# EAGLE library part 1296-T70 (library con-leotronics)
1.27mm SINGLE ROW FEMALE SOCKET Source: http://www.leotronics.co.uk/Conexcon/Data%20Sheets/sec.%20A/1296ing.pdf
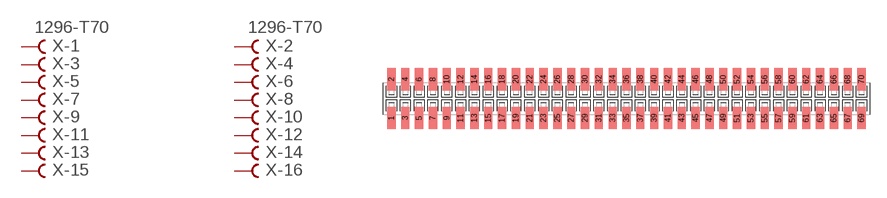
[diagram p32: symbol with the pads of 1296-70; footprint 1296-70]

Designator prefix X; gates -1=FVAL -2=FVAL -3=F -4=F -5=F -6=F -7=F -8=F -9=F -10=F -11=F -12=F -13=F -14=F -15=F -16=F -17=F -18=F -19=F -20=F -21=F -22=F -23=F -24=F -25=F -26=F -27=F -28=F -29=F -30=F -31=F -32=F -33=F -34=F -35=F -36=F -37=F -38=F -39=F -40=F -41=F -42=F -43=F -44=F -45=F -46=F -47=F -48=F -49=F -50=F -51=F -52=F -53=F -54=F -55=F -56=F -57=F -58=F -59=F -60=F -61=F -62=F -63=F -64=F -65=F -66=F -67=F -68=F -69=F -70=F

## 1296-T70 (OC_FARNELL: unknown; OC_NEWARK: unknown)  [1296-70]
1  -1:B  pas
2  -2:B  pas
3  -3:B  pas
4  -4:B  pas
5  -5:B  pas
6  -6:B  pas
7  -7:B  pas
8  -8:B  pas
9  -9:B  pas
10  -10:B  pas
11  -11:B  pas
12  -12:B  pas
13  -13:B  pas
14  -14:B  pas
15  -15:B  pas
16  -16:B  pas
17  -17:B  pas
18  -18:B  pas
19  -19:B  pas
20  -20:B  pas
21  -21:B  pas
22  -22:B  pas
23  -23:B  pas
24  -24:B  pas
25  -25:B  pas
26  -26:B  pas
27  -27:B  pas
28  -28:B  pas
29  -29:B  pas
30  -30:B  pas
31  -31:B  pas
32  -32:B  pas
33  -33:B  pas
34  -34:B  pas
35  -35:B  pas
36  -36:B  pas
37  -37:B  pas
38  -38:B  pas
39  -39:B  pas
40  -40:B  pas
41  -41:B  pas
42  -42:B  pas
43  -43:B  pas
44  -44:B  pas
45  -45:B  pas
46  -46:B  pas
47  -47:B  pas
48  -48:B  pas
49  -49:B  pas
50  -50:B  pas
51  -51:B  pas
52  -52:B  pas
53  -53:B  pas
54  -54:B  pas
55  -55:B  pas
56  -56:B  pas
57  -57:B  pas
58  -58:B  pas
59  -59:B  pas
60  -60:B  pas
61  -61:B  pas
62  -62:B  pas
63  -63:B  pas
64  -64:B  pas
65  -65:B  pas
66  -66:B  pas
67  -67:B  pas
68  -68:B  pas
69  -69:B  pas
70  -70:B  pas

## Footprint 1296-70 (pad centres in mm)
1.27mm SINGLE ROW FEMALE SOCKET Source: http://www.leotronics.co.uk/Conexcon/Data%20Sheets/sec.%20A/1296ing.pdf
smd 0.76 x 2.05: 1 -21.59,-1.78; 2 -21.59,1.78; 3 -20.32,-1.78; 4 -20.32,1.78; 5 -19.05,-1.78; 6 -19.05,1.78; 7 -17.78,-1.78; 8 -17.78,1.78; 9 -16.51,-1.78; 10 -16.51,1.78; 11 -15.24,-1.78; 12 -15.24,1.78; 13 -13.97,-1.78; 14 -13.97,1.78; 15 -12.7,-1.78; 16 -12.7,1.78; 17 -11.43,-1.78; 18 -11.43,1.78; 19 -10.16,-1.78; 20 -10.16,1.78; 21 -8.89,-1.78; 22 -8.89,1.78; 23 -7.62,-1.78; 24 -7.62,1.78; 25 -6.35,-1.78; 26 -6.35,1.78; 27 -5.08,-1.78; 28 -5.08,1.78; 29 -3.81,-1.78; 30 -3.81,1.78; 31 -2.54,-1.78; 32 -2.54,1.78; 33 -1.27,-1.78; 34 -1.27,1.78; 35 0,-1.78; 36 0,1.78; 37 1.27,-1.78; 38 1.27,1.78; 39 2.54,-1.78; 40 2.54,1.78; 41 3.81,-1.78; 42 3.81,1.78; 43 5.08,-1.78; 44 5.08,1.78; 45 6.35,-1.78; 46 6.35,1.78; 47 7.62,-1.78; 48 7.62,1.78; 49 8.89,-1.78; 50 8.89,1.78; 51 10.16,-1.78; 52 10.16,1.78; 53 11.43,-1.78; 54 11.43,1.78; 55 12.7,-1.78; 56 12.7,1.78; 57 13.97,-1.78; 58 13.97,1.78; 59 15.24,-1.78; 60 15.24,1.78; 61 16.51,-1.78; 62 16.51,1.78; 63 17.78,-1.78; 64 17.78,1.78; 65 19.05,-1.78; 66 19.05,1.78; 67 20.32,-1.78; 68 20.32,1.78; 69 21.59,-1.78; 70 21.59,1.78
